(* Logix 5000 AddOnInstructionDefinition export IOLService; software revision 19.01 *)

TYPE IOLRequest :
STRUCT
   Enable_Multiple_Nodes : BOOL; {access None}   // Set to 1 to enable multiple nodes
   ApplicationPath : STRING; {access None}   // Set Path for following IOL Instructions
   Read : BOOL; {access None}   // For internal use to integrate IOLRead and IOWrite with IOLService
   Write : BOOL; {access None}   // For internal use to integrate IOLRead and IOWrite with IOLService
   Reset : BOOL; {access None}   // For internal use to integrate IOLRead and IOWrite with IOLService
   Done : BOOL; {access None}   // For internal use to integrate IOLRead and IOWrite with IOLService
   Error : BOOL; {access None}   // For internal use to integrate IOLRead and IOWrite with IOLService
   Slot : INT; {access None}   // For internal use to integrate IOLRead and IOWrite with IOLService
   Port : INT; {access None}   // For internal use to integrate IOLRead and IOWrite with IOLService
   Index : INT; {access None}   // For internal use to integrate IOLRead and IOWrite with IOLService
   SubIndex : INT; {access None}   // For internal use to integrate IOLRead and IOWrite with IOLService
   Length : INT; {access None}   // For internal use to integrate IOLRead and IOWrite with IOLService
   Handle : INT; {access None}   // For internal use to integrate IOLRead and IOWrite with IOLService
   Status : INT; {access None}   // For internal use to integrate IOLRead and IOWrite with IOLService
   NextHandle : INT; {access None}   // For internal use to integrate IOLRead and IOWrite with IOLService
   ReceiveData : SINT[145]; {access None}   // For internal use to integrate IOLRead and IOWrite with IOLService
   SendData : SINT[145]; {access None}   // For internal use to integrate IOLRead and IOWrite with IOLService
   WriteData : DINT; {access None}   // For internal use to integrate IOLRead and IOWrite with IOLService
   ActivePath : STRING; {access None}   // For internal use to integrate IOLRead and IOWrite with IOLService
END_STRUCT
END_TYPE

ADD_ON_INSTRUCTION IOLService   (* revision 1.2, ExecutePrescan *)
// Revision note:
// V1_0 Initial Release
// V1_1 Added error checking for IOLWrite operations
// V1_2 Added multiple EIP node support
// Help:
// IOL_Service - used with Turck BL20, BL67, BLC and TBEN IOLink masters to process requests from IOL_ReadString, IOL_WriteString, IOL_ReadData and IOL_WriteData AOI's.
// Status	Description
// 0	Operation completed successfully
// 	Status = 100 - 102, Ethernet IP MSG instruction errors - check communication parameters
// 100	IOL_SendMSG completed with error, check communication parameters
// 101	IOL_RecevieMSG completed with error, check communication parameters
// 110	IOL_Service Retry Limit exceeded
// 111	Slot specified not an IOLink master
// 	Status = 1000 to 1255, no response from device, connection error
// 1016	Device not connected or Port not configured as IOLink port
// 	Status = 2000 to 2255,  device response indicates error
// 2000	Device error, no details
// 2017	Device error, Index not available
// 2018	Device error, Subindex not available
// 2032	Device error, Service temporarily not available
// 2033	Device error, Service temporarily not available - local control
// 2034	Device error, Service temporarily not available - device control
// 2035	Device error, Index not writeable
// 2048	Device error, Parameter value out of range
// 2049	Device error, Parameter value above limit
// 2050	Device error, Parameter value below limit
// 2051	Device error, Parameter value length overrun (check IOLWrite precision/string length)
// 2052	Device error, Parameter value length underrun (check IOLWrite precision/string length)
// 2053	Device error, Function not available
// 2054	Device error, Function temporarily not available
// 2064	Device error, Parameter set invalid
// 2065	Device error, Inconsistent parameter set
// 2130	Device error, Application not ready
// 	Status = 3000 to 3255,   device response indicates vendor specific error
// 3000	Vendor specific error, no details
// 3001	Vendor specific error, vendor specific error number
// 3255	Vendor specific error, vendor specific error number
// 	Status = 7000 to 7255,  IOL-M Error Codes
// 7000	Unexpected write request instead of read request
// 7001	Decode error
// 7002	Port occupied by another task
// 	Status = 8000 to 8255,  IOL-M Error Codes
// 8000	Timeout when IOL-Ds or IOL-M ports are busy
// 8001	IOL Index out of range
// 8002	Port address greater than maximum
// 8003	Port function not supported
VAR_IN_OUT
   IOLData : IOLRequest; {required}
   IOL_SendMSG : MESSAGE; {required}
   IOL_ReceiveMSG : MESSAGE; {required}
END_VAR
VAR
   IOLS1 : BOOL;
   IOLS2 : BOOL;
   IOLS3 : BOOL;
   IOLS4 : BOOL;
   IOLS5 : BOOL;
   IOLS6 : BOOL;
   IOLS7 : BOOL;
   IOLReadActive : BOOL;
   IOLWriteActive : BOOL;
   Retry : BOOL;
   RetryCount : DINT;
   IOL_SendMSG_Request : BOOL; {access None}
   IOL_ReceiveMSG_Request : BOOL; {access None}
   IOLS4_Bad : BOOL; {access None}
   IOL_S2_0_Count : DINT; {access None}
   IOL_S6_0_Count : DINT; {access None}
   Busy_Retry : BOOL; {access None}
   IOL_S2_0_Total : DINT; {access None}
   IOL_S3_Retry : DINT; {access None}
   IOL_S1_Count : DINT; {access None}
   IOL_S2_Count : DINT; {access None}
   IOL_S3_Count : DINT; {access None}
   IOL_S5_Count : DINT; {access None}
   IOL_S6_Count : DINT; {access None}
   ER1 : BOOL; {access None}
   ER2 : BOOL; {access None}
   IOL_S6_NotBusy_Count : DINT; {access None}
   RetryTotal : DINT; {access None}
   IOL_S4_Bad_Count : DINT; {access None}
   IOL_S2_Error_Count : DINT; {access None}
   IOL_Done_Count : DINT; {access None}
   IOL_Error_Count : DINT; {access None}
   IOLReset_ONS : BOOL; {access None}
   ABS_RD_11 : INT; {access None}
   ABS_RD_12 : INT; {access None}
   ABS_RD_13 : INT; {access None}
   IOL_SendMSG_DN : BOOL; {access None}
   IOL_ReceiveMSG_DN : BOOL; {access None}
   IOLS2A : BOOL; {access None}
   Generate_Status : BOOL; {access None}
   IOLS5A : BOOL; {access None}
   Busy_Response : BOOL; {access None}
   Done_Response : BOOL; {access None}
   IOL_S6_Done_Count : DINT; {access None}
   Wait : BOOL; {access None}
   IOL_S6_Busy_Count : DINT; {access None}
END_VAR

ROUTINE Logic   (* ladder *)
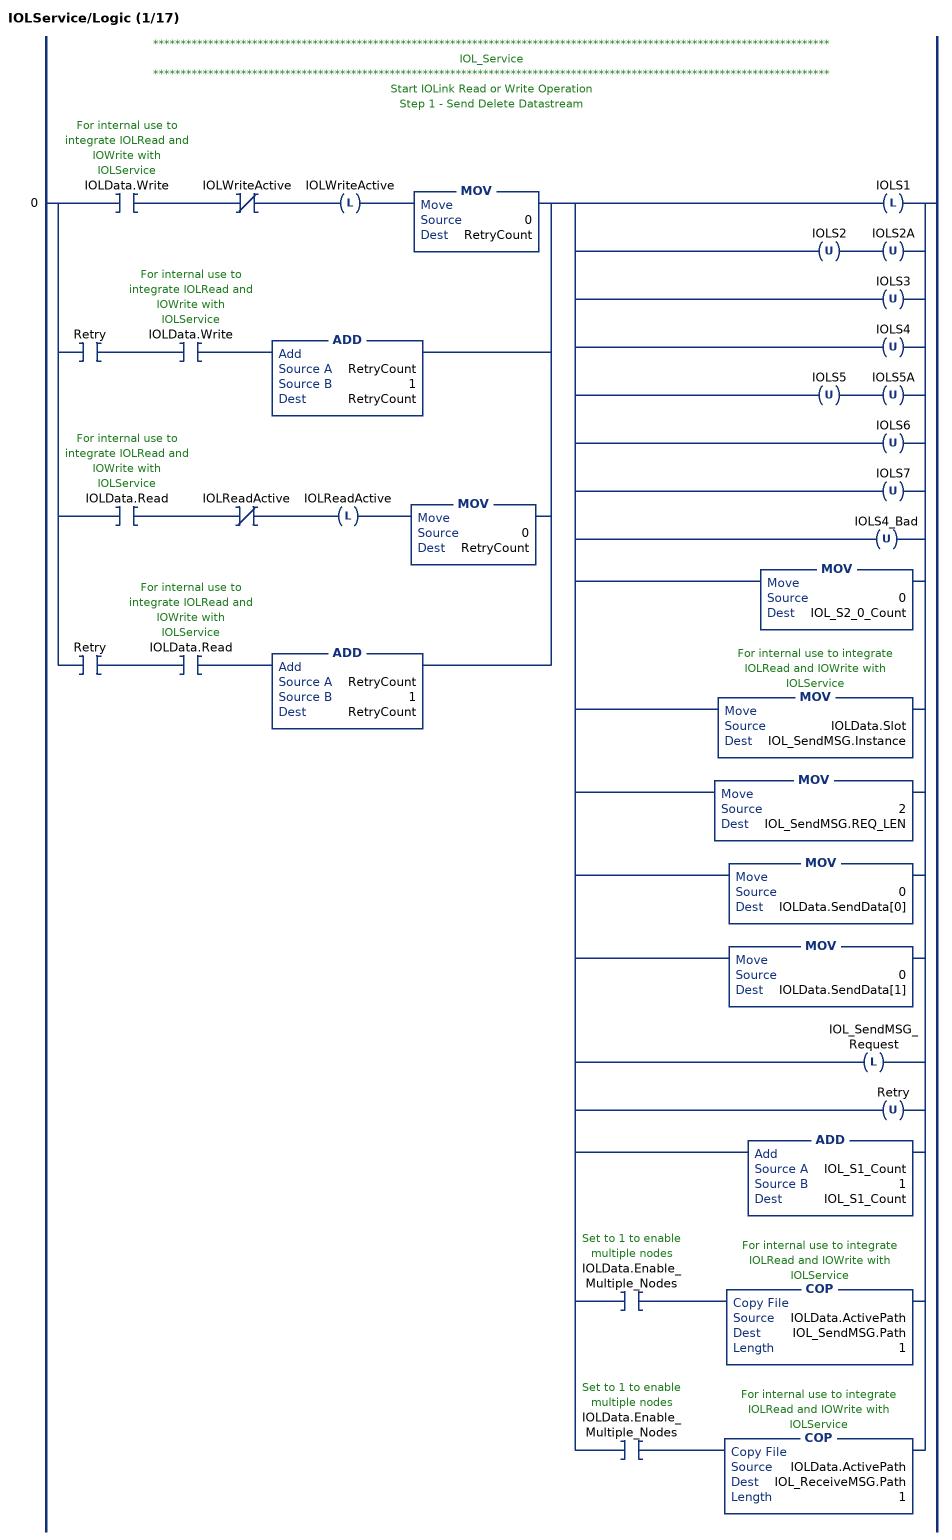
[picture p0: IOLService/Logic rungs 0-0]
   // ***************************************************************************************************************************
   // IOL_Service
   // ***************************************************************************************************************************
   // Start IOLink Read or Write Operation
   // Step 1 - Send Delete Datastream
   0: [XIC(IOLData.Write) XIO(IOLWriteActive) OTL(IOLWriteActive) MOV(0,RetryCount) ,XIC(Retry) XIC(IOLData.Write) ADD(RetryCount,1,RetryCount) ,XIC(IOLData.Read) XIO(IOLReadActive) OTL(IOLReadActive) MOV(0,RetryCount) ,XIC(Retry) XIC(IOLData.Read) ADD(RetryCount,1,RetryCount) ][OTL(IOLS1) ,OTU(IOLS2) OTU(IOLS2A) ,OTU(IOLS3) ,OTU(IOLS4) ,OTU(IOLS5) OTU(IOLS5A) ,OTU(IOLS6) ,OTU(IOLS7) ,OTU(IOLS4_Bad) ,MOV(0,IOL_S2_0_Count) ,MOV(IOLData.Slot,IOL_SendMSG.Instance) ,MOV(2,IOL_SendMSG.REQ_LEN) ,MOV(0,IOLData.SendData[0]) ,MOV(0,IOLData.SendData[1]) ,OTL(IOL_SendMSG_Request) ,OTU(Retry) ,ADD(IOL_S1_Count,1,IOL_S1_Count) ,XIC(IOLData.Enable_Multiple_Nodes) COP(IOLData.ActivePath,IOL_SendMSG.Path,1) ,XIC(IOLData.Enable_Multiple_Nodes) COP(IOLData.ActivePath,IOL_ReceiveMSG.Path,1) ];
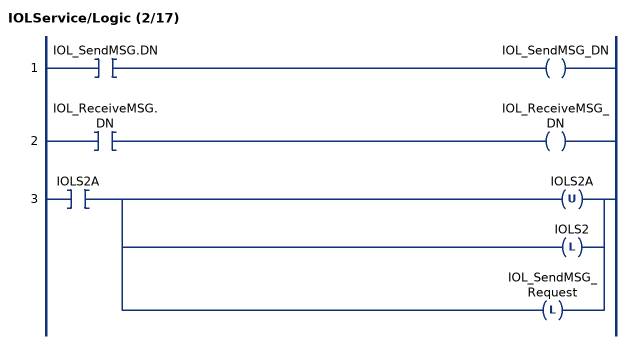
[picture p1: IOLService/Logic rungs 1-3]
   1: XIC(IOL_SendMSG.DN)OTE(IOL_SendMSG_DN);
   2: XIC(IOL_ReceiveMSG.DN)OTE(IOL_ReceiveMSG_DN);
   3: XIC(IOLS2A)[OTU(IOLS2A) ,OTL(IOLS2) ,OTL(IOL_SendMSG_Request) ];
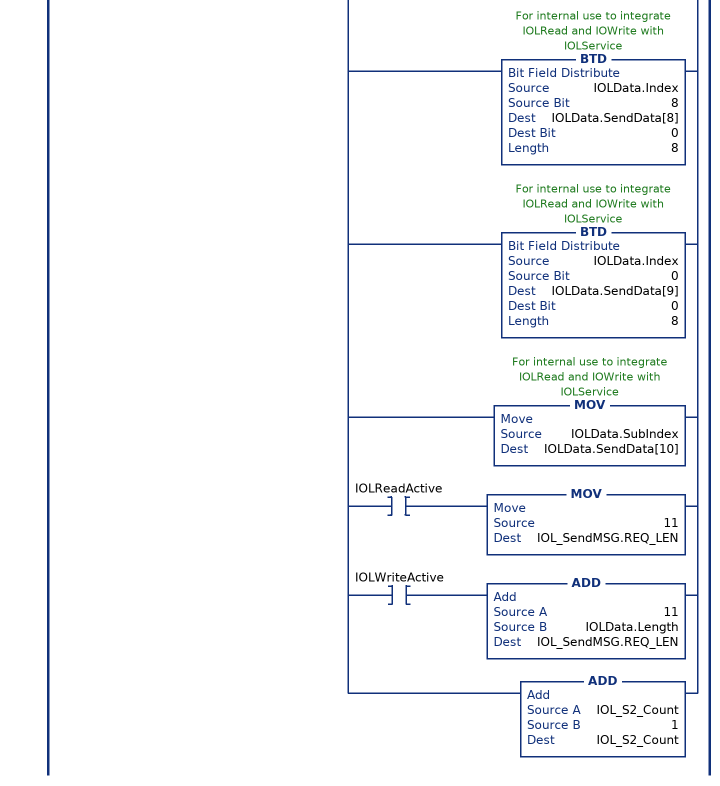
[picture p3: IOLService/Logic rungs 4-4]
   // Step 1 - After Delete Stream sent then Send IOLink Read or Write Request
   4: XIC(IOLS1)XIC(IOL_SendMSG_DN)XIO(IOL_SendMSG_Request)[OTU(IOLS1) ,OTL(IOLS2A) ,MOV(IOLData.Slot,IOL_SendMSG.Instance) ,MOV(0,IOLData.SendData[0]) ,MOV(16#fe,IOLData.SendData[1]) ,MOV(16#11,IOLData.SendData[2]) ,MOV(16#08,IOLData.SendData[3]) ,MOV(IOLData.Port,IOLData.SendData[4]) ,MOV(16#fe,IOLData.SendData[5]) ,MOV(16#4a,IOLData.SendData[6]) ,XIC(IOLReadActive) MOV(16#03,IOLData.SendData[7]) ,XIC(IOLWriteActive) MOV(16#02,IOLData.SendData[7]) ,BTD(IOLData.Index,8,IOLData.SendData[8],0,8) ,BTD(IOLData.Index,0,IOLData.SendData[9],0,8) ,MOV(IOLData.SubIndex,IOLData.SendData[10]) ,XIC(IOLReadActive) MOV(11,IOL_SendMSG.REQ_LEN) ,XIC(IOLWriteActive) ADD(11,IOLData.Length,IOL_SendMSG.REQ_LEN) ,ADD(IOL_S2_Count,1,IOL_S2_Count) ];
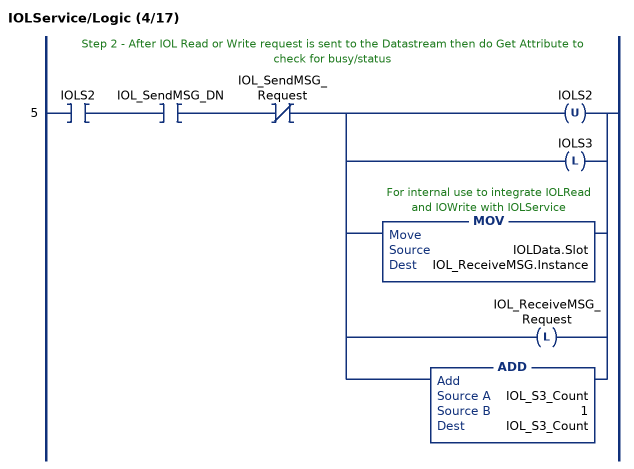
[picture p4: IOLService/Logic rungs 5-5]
   // Step 2 - After IOL Read or Write request is sent to the Datastream then do Get Attribute to check for busy/status
   5: XIC(IOLS2)XIC(IOL_SendMSG_DN)XIO(IOL_SendMSG_Request)[OTU(IOLS2) ,OTL(IOLS3) ,MOV(IOLData.Slot,IOL_ReceiveMSG.Instance) ,OTL(IOL_ReceiveMSG_Request) ,ADD(IOL_S3_Count,1,IOL_S3_Count) ];
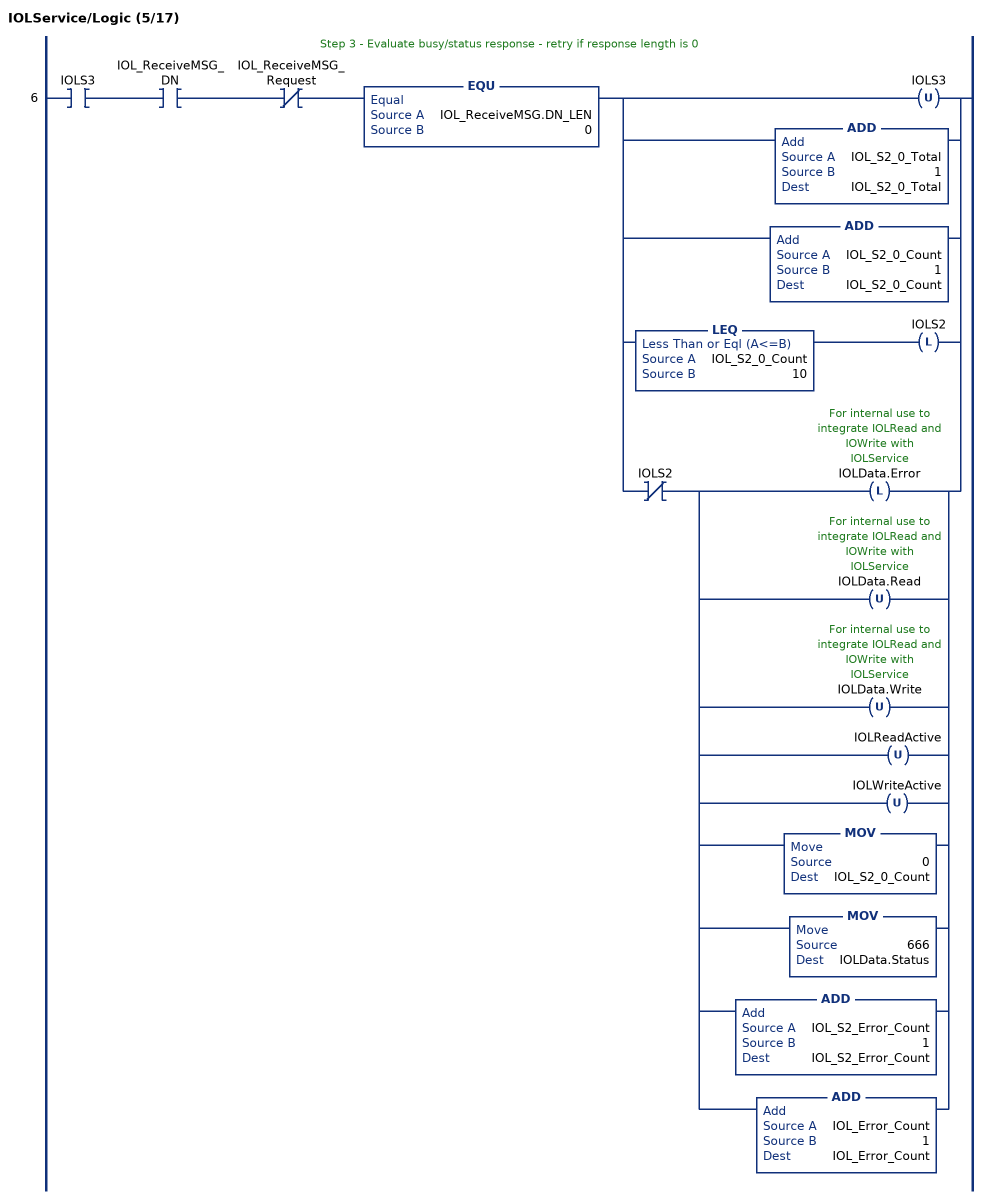
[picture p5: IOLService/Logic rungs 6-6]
   // Step 3 - Evaluate busy/status response - retry if response length is 0
   6: XIC(IOLS3)XIC(IOL_ReceiveMSG_DN)XIO(IOL_ReceiveMSG_Request)EQU(IOL_ReceiveMSG.DN_LEN,0)[OTU(IOLS3) ,ADD(IOL_S2_0_Total,1,IOL_S2_0_Total) ,ADD(IOL_S2_0_Count,1,IOL_S2_0_Count) ,LEQ(IOL_S2_0_Count,10) OTL(IOLS2) ,XIO(IOLS2) [OTL(IOLData.Error) ,OTU(IOLData.Read) ,OTU(IOLData.Write) ,OTU(IOLReadActive) ,OTU(IOLWriteActive) ,MOV(0,IOL_S2_0_Count) ,MOV(666,IOLData.Status) ,ADD(IOL_S2_Error_Count,1,IOL_S2_Error_Count) ,ADD(IOL_Error_Count,1,IOL_Error_Count) ] ];
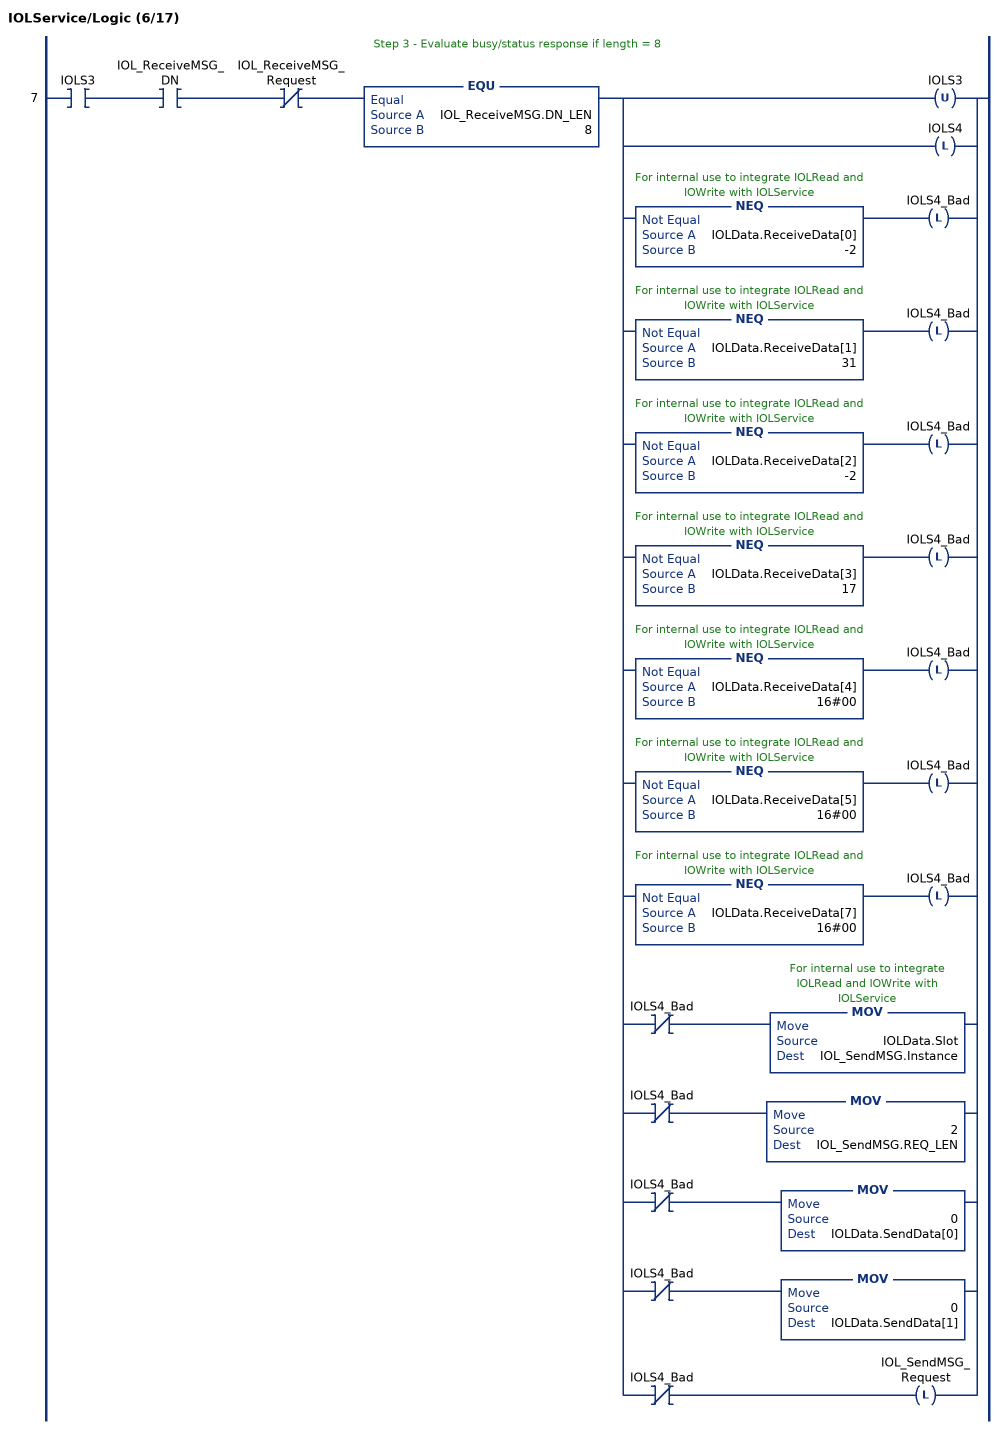
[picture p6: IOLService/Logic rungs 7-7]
   // Step 3 - Evaluate busy/status response if length = 8
   7: XIC(IOLS3)XIC(IOL_ReceiveMSG_DN)XIO(IOL_ReceiveMSG_Request)EQU(IOL_ReceiveMSG.DN_LEN,8)[OTU(IOLS3) ,OTL(IOLS4) ,NEQ(IOLData.ReceiveData[0],-2) OTL(IOLS4_Bad) ,NEQ(IOLData.ReceiveData[1],31) OTL(IOLS4_Bad) ,NEQ(IOLData.ReceiveData[2],-2) OTL(IOLS4_Bad) ,NEQ(IOLData.ReceiveData[3],17) OTL(IOLS4_Bad) ,NEQ(IOLData.ReceiveData[4],16#00) OTL(IOLS4_Bad) ,NEQ(IOLData.ReceiveData[5],16#00) OTL(IOLS4_Bad) ,NEQ(IOLData.ReceiveData[7],16#00) OTL(IOLS4_Bad) ,XIO(IOLS4_Bad) MOV(IOLData.Slot,IOL_SendMSG.Instance) ,XIO(IOLS4_Bad) MOV(2,IOL_SendMSG.REQ_LEN) ,XIO(IOLS4_Bad) MOV(0,IOLData.SendData[0]) ,XIO(IOLS4_Bad) MOV(0,IOLData.SendData[1]) ,XIO(IOLS4_Bad) OTL(IOL_SendMSG_Request) ];
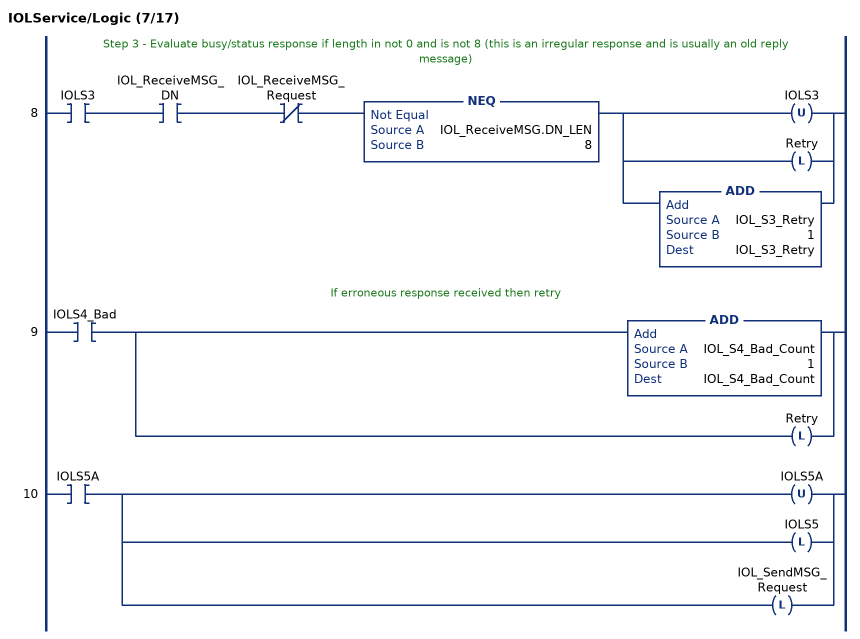
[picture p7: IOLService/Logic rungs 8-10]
   // Step 3 - Evaluate busy/status response if length in not 0 and is not 8 (this is an irregular response and is usually an old reply message)
   8: XIC(IOLS3)XIC(IOL_ReceiveMSG_DN)XIO(IOL_ReceiveMSG_Request)NEQ(IOL_ReceiveMSG.DN_LEN,8)[OTU(IOLS3) ,OTL(Retry) ,ADD(IOL_S3_Retry,1,IOL_S3_Retry) ];
   // If erroneous response received then retry
   9: XIC(IOLS4_Bad)[ADD(IOL_S4_Bad_Count,1,IOL_S4_Bad_Count) ,OTL(Retry) ];
   10: XIC(IOLS5A)[OTU(IOLS5A) ,OTL(IOLS5) ,OTL(IOL_SendMSG_Request) ];
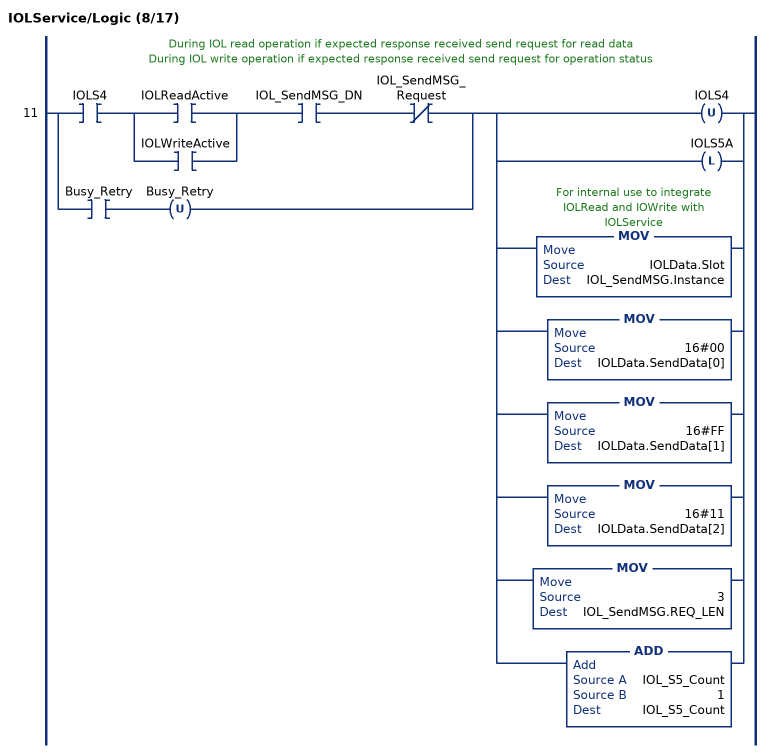
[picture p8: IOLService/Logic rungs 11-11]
   // During IOL read operation if expected response received send request for read data
   // During IOL write operation if expected response received send request for operation status
   11: [XIC(IOLS4) [XIC(IOLReadActive) ,XIC(IOLWriteActive) ] XIC(IOL_SendMSG_DN) XIO(IOL_SendMSG_Request) ,XIC(Busy_Retry) OTU(Busy_Retry) ][OTU(IOLS4) ,OTL(IOLS5A) ,MOV(IOLData.Slot,IOL_SendMSG.Instance) ,MOV(16#00,IOLData.SendData[0]) ,MOV(16#FF,IOLData.SendData[1]) ,MOV(16#11,IOLData.SendData[2]) ,MOV(3,IOL_SendMSG.REQ_LEN) ,ADD(IOL_S5_Count,1,IOL_S5_Count) ];
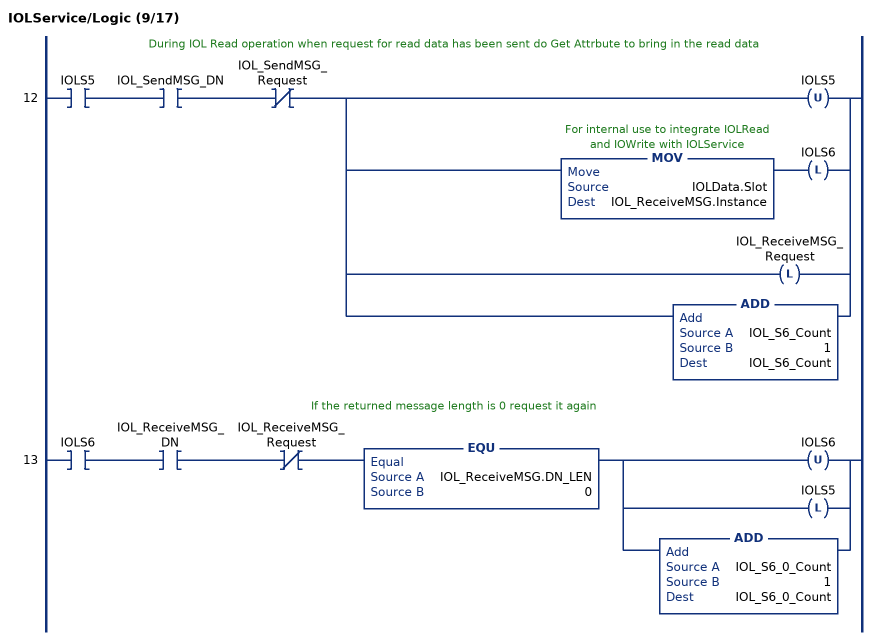
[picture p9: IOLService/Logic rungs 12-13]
   // During IOL Read operation when request for read data has been sent do Get Attrbute to bring in the read data
   12: XIC(IOLS5)XIC(IOL_SendMSG_DN)XIO(IOL_SendMSG_Request)[OTU(IOLS5) ,MOV(IOLData.Slot,IOL_ReceiveMSG.Instance) OTL(IOLS6) ,OTL(IOL_ReceiveMSG_Request) ,ADD(IOL_S6_Count,1,IOL_S6_Count) ];
   // If the returned message length is 0 request it again
   13: XIC(IOLS6)XIC(IOL_ReceiveMSG_DN)XIO(IOL_ReceiveMSG_Request)EQU(IOL_ReceiveMSG.DN_LEN,0)[OTU(IOLS6) ,OTL(IOLS5) ,ADD(IOL_S6_0_Count,1,IOL_S6_0_Count) ];
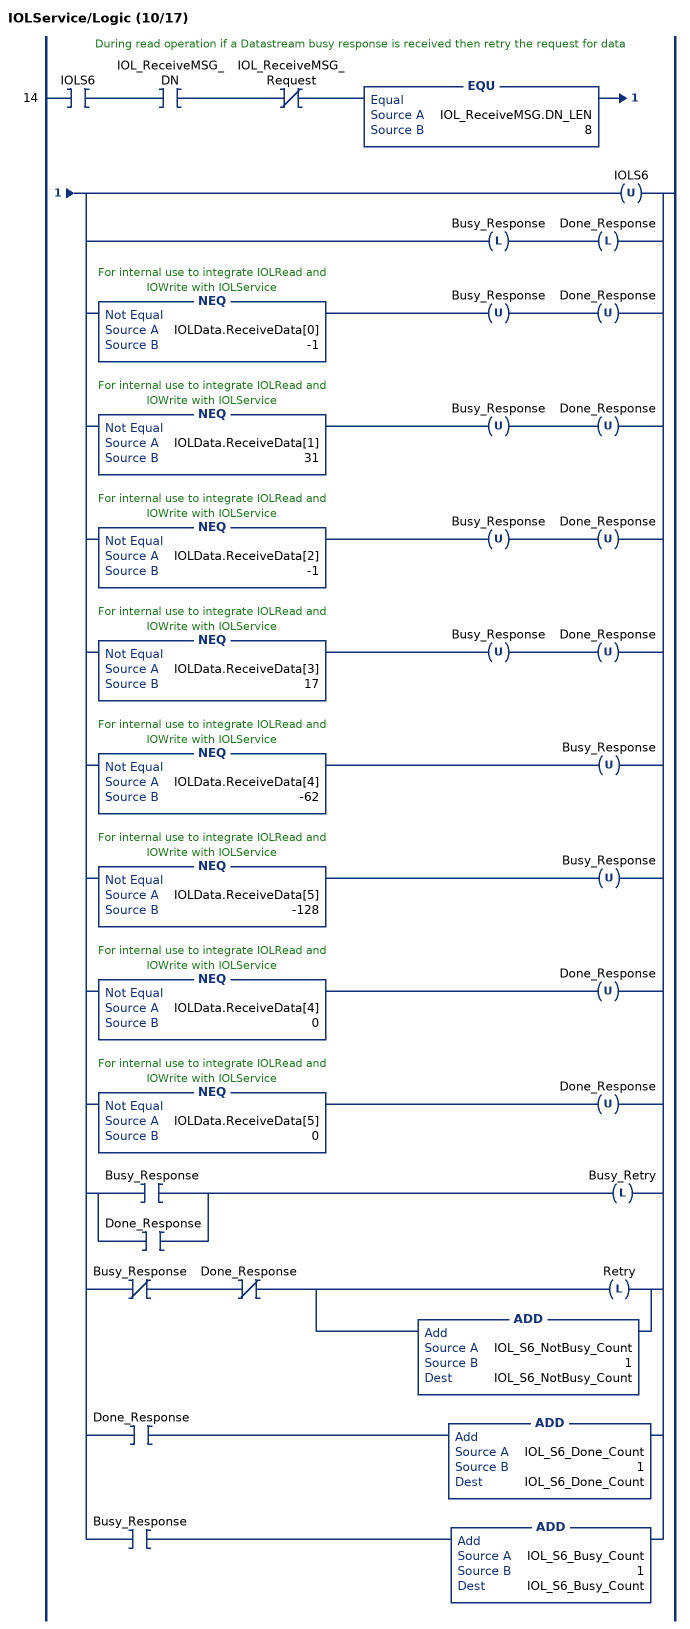
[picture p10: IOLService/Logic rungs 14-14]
   // During read operation if a Datastream busy response is received then retry the request for data
   14: XIC(IOLS6)XIC(IOL_ReceiveMSG_DN)XIO(IOL_ReceiveMSG_Request)EQU(IOL_ReceiveMSG.DN_LEN,8)[OTU(IOLS6) ,OTL(Busy_Response) OTL(Done_Response) ,NEQ(IOLData.ReceiveData[0],-1) OTU(Busy_Response) OTU(Done_Response) ,NEQ(IOLData.ReceiveData[1],31) OTU(Busy_Response) OTU(Done_Response) ,NEQ(IOLData.ReceiveData[2],-1) OTU(Busy_Response) OTU(Done_Response) ,NEQ(IOLData.ReceiveData[3],17) OTU(Busy_Response) OTU(Done_Response) ,NEQ(IOLData.ReceiveData[4],-62) OTU(Busy_Response) ,NEQ(IOLData.ReceiveData[5],-128) OTU(Busy_Response) ,NEQ(IOLData.ReceiveData[4],0) OTU(Done_Response) ,NEQ(IOLData.ReceiveData[5],0) OTU(Done_Response) ,[XIC(Busy_Response) ,XIC(Done_Response) ] OTL(Busy_Retry) ,XIO(Busy_Response) XIO(Done_Response) [OTL(Retry) ,ADD(IOL_S6_NotBusy_Count,1,IOL_S6_NotBusy_Count) ] ,XIC(Done_Response) ADD(IOL_S6_Done_Count,1,IOL_S6_Done_Count) ,XIC(Busy_Response) ADD(IOL_S6_Busy_Count,1,IOL_S6_Busy_Count) ];
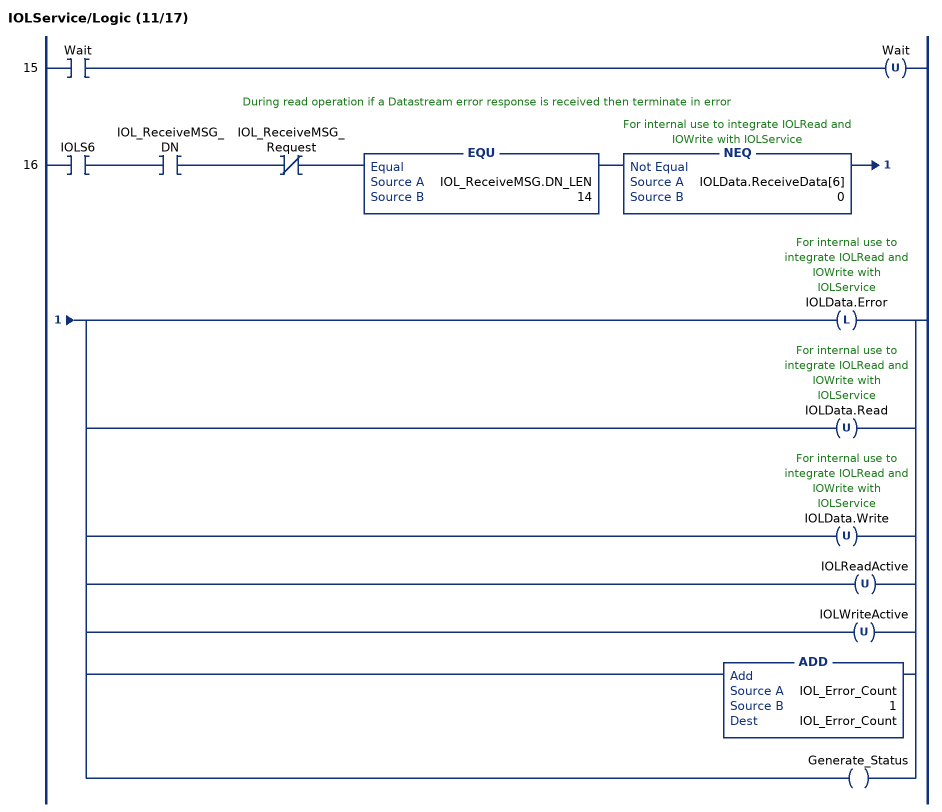
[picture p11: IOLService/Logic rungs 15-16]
   15: XIC(Wait)OTU(Wait);
   // During read operation if a Datastream error response is received then terminate in error
   16: XIC(IOLS6)XIC(IOL_ReceiveMSG_DN)XIO(IOL_ReceiveMSG_Request)EQU(IOL_ReceiveMSG.DN_LEN,14)NEQ(IOLData.ReceiveData[6],0)[OTL(IOLData.Error) ,OTU(IOLData.Read) ,OTU(IOLData.Write) ,OTU(IOLReadActive) ,OTU(IOLWriteActive) ,ADD(IOL_Error_Count,1,IOL_Error_Count) ,OTE(Generate_Status) ];
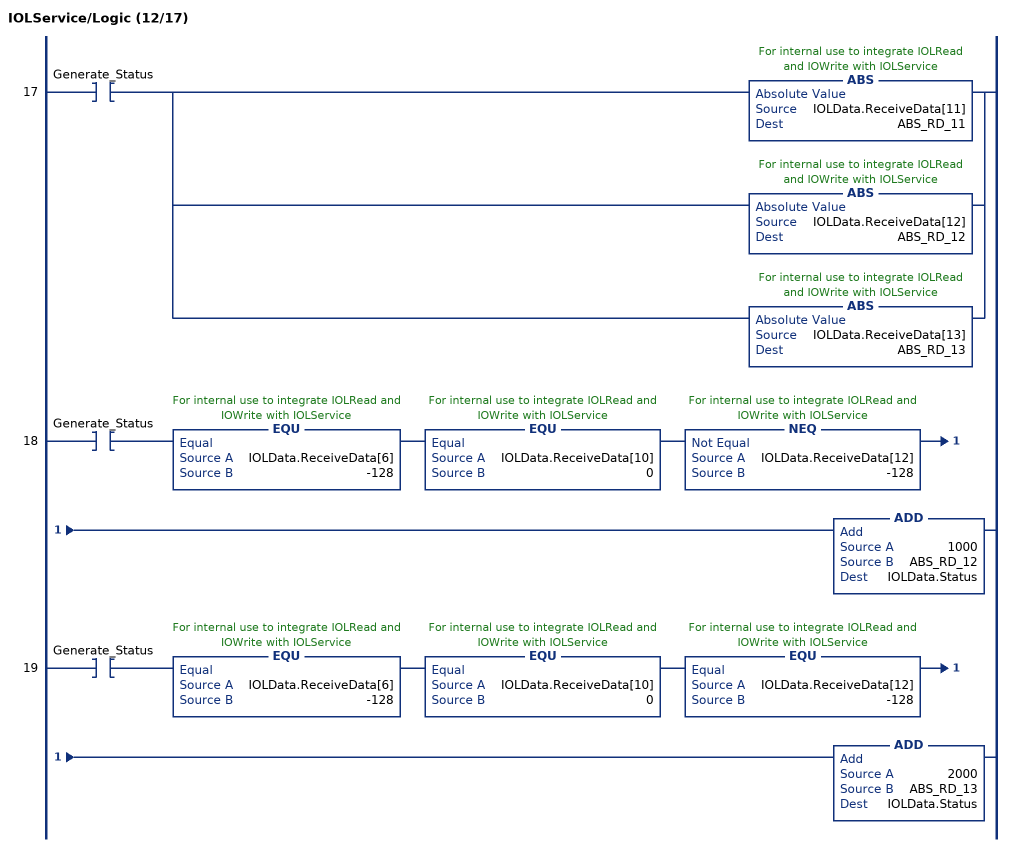
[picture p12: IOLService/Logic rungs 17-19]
   17: XIC(Generate_Status)[ABS(IOLData.ReceiveData[11],ABS_RD_11) ,ABS(IOLData.ReceiveData[12],ABS_RD_12) ,ABS(IOLData.ReceiveData[13],ABS_RD_13) ];
   18: XIC(Generate_Status)EQU(IOLData.ReceiveData[6],-128)EQU(IOLData.ReceiveData[10],0)NEQ(IOLData.ReceiveData[12],-128)ADD(1000,ABS_RD_12,IOLData.Status);
   19: XIC(Generate_Status)EQU(IOLData.ReceiveData[6],-128)EQU(IOLData.ReceiveData[10],0)EQU(IOLData.ReceiveData[12],-128)ADD(2000,ABS_RD_13,IOLData.Status);
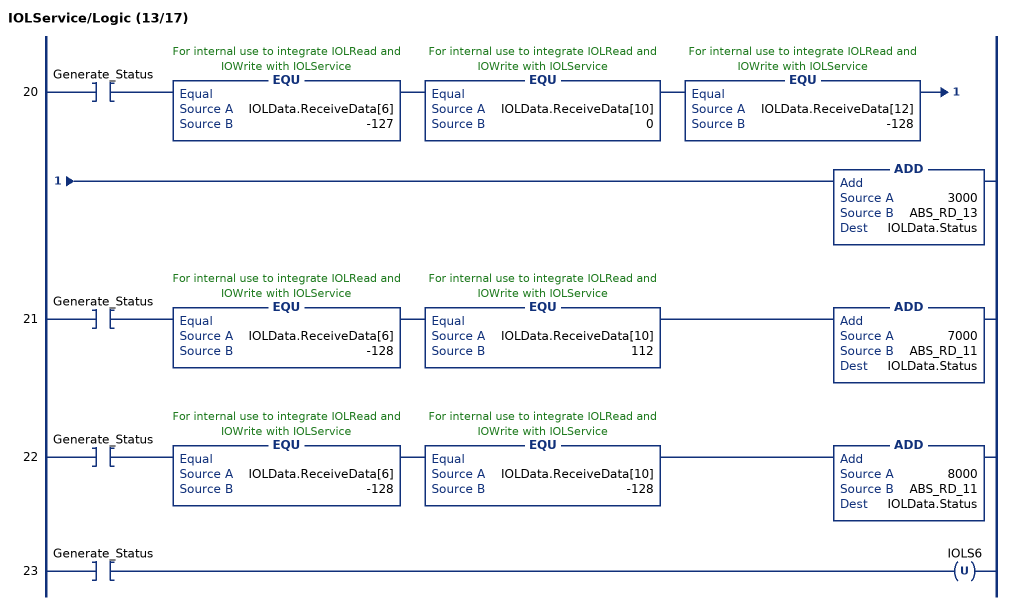
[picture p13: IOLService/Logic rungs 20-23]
   20: XIC(Generate_Status)EQU(IOLData.ReceiveData[6],-127)EQU(IOLData.ReceiveData[10],0)EQU(IOLData.ReceiveData[12],-128)ADD(3000,ABS_RD_13,IOLData.Status);
   21: XIC(Generate_Status)EQU(IOLData.ReceiveData[6],-128)EQU(IOLData.ReceiveData[10],112)ADD(7000,ABS_RD_11,IOLData.Status);
   22: XIC(Generate_Status)EQU(IOLData.ReceiveData[6],-128)EQU(IOLData.ReceiveData[10],-128)ADD(8000,ABS_RD_11,IOLData.Status);
   23: XIC(Generate_Status)OTU(IOLS6);
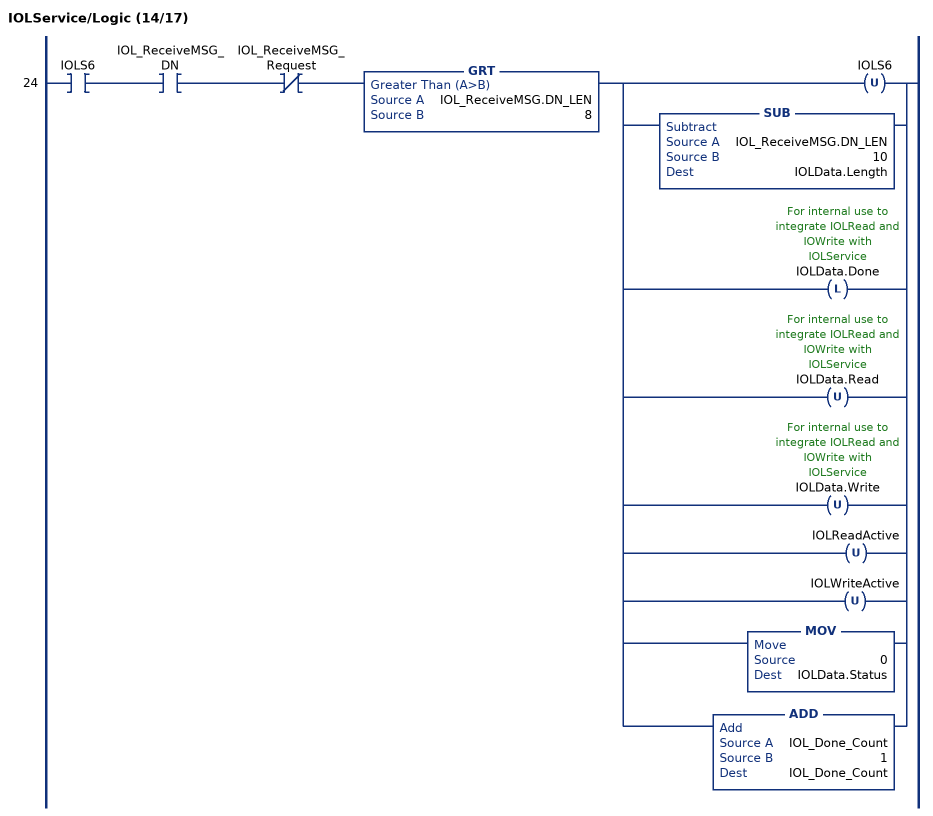
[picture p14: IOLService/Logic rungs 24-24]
   24: XIC(IOLS6)XIC(IOL_ReceiveMSG_DN)XIO(IOL_ReceiveMSG_Request)GRT(IOL_ReceiveMSG.DN_LEN,8)[OTU(IOLS6) ,SUB(IOL_ReceiveMSG.DN_LEN,10,IOLData.Length) ,OTL(IOLData.Done) ,OTU(IOLData.Read) ,OTU(IOLData.Write) ,OTU(IOLReadActive) ,OTU(IOLWriteActive) ,MOV(0,IOLData.Status) ,ADD(IOL_Done_Count,1,IOL_Done_Count) ];
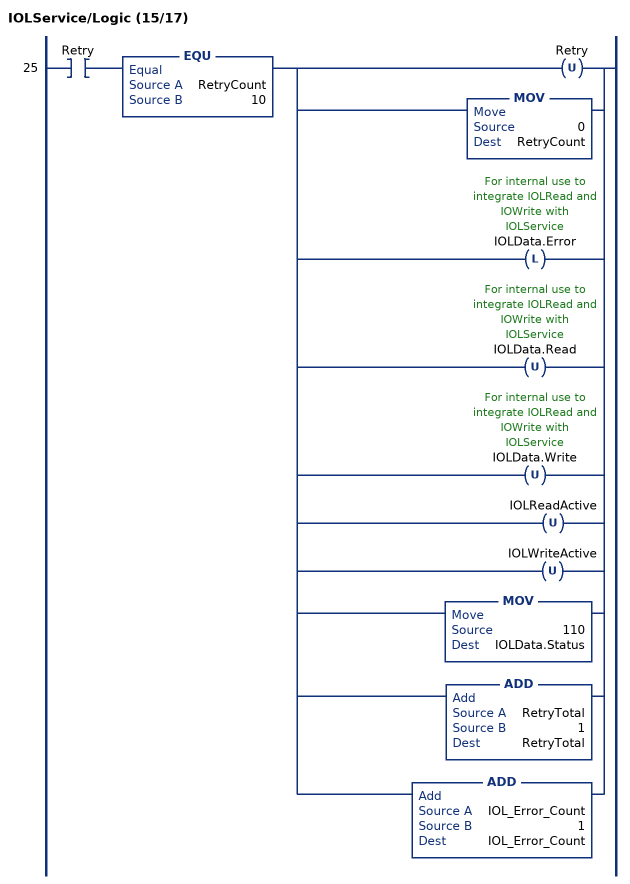
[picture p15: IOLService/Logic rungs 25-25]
   25: XIC(Retry)EQU(RetryCount,10)[OTU(Retry) ,MOV(0,RetryCount) ,OTL(IOLData.Error) ,OTU(IOLData.Read) ,OTU(IOLData.Write) ,OTU(IOLReadActive) ,OTU(IOLWriteActive) ,MOV(110,IOLData.Status) ,ADD(RetryTotal,1,RetryTotal) ,ADD(IOL_Error_Count,1,IOL_Error_Count) ];
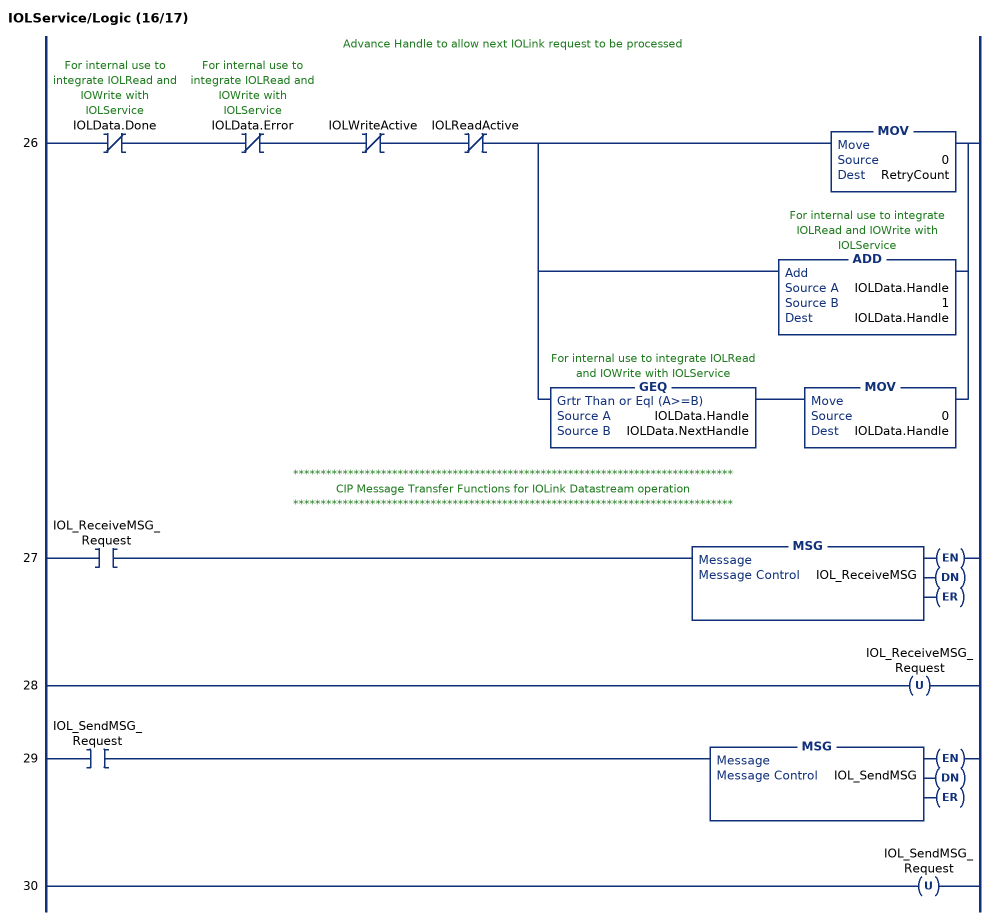
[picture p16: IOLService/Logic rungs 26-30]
   // Advance Handle to allow next IOLink request to be processed
   26: XIO(IOLData.Done)XIO(IOLData.Error)XIO(IOLWriteActive)XIO(IOLReadActive)[MOV(0,RetryCount) ,ADD(IOLData.Handle,1,IOLData.Handle) ,GEQ(IOLData.Handle,IOLData.NextHandle) MOV(0,IOLData.Handle) ];
   // ********************************************************************************
   // CIP Message Transfer Functions for IOLink Datastream operation
   // ********************************************************************************
   27: XIC(IOL_ReceiveMSG_Request)MSG(IOL_ReceiveMSG);
   28: OTU(IOL_ReceiveMSG_Request);
   29: XIC(IOL_SendMSG_Request)MSG(IOL_SendMSG);
   30: OTU(IOL_SendMSG_Request);
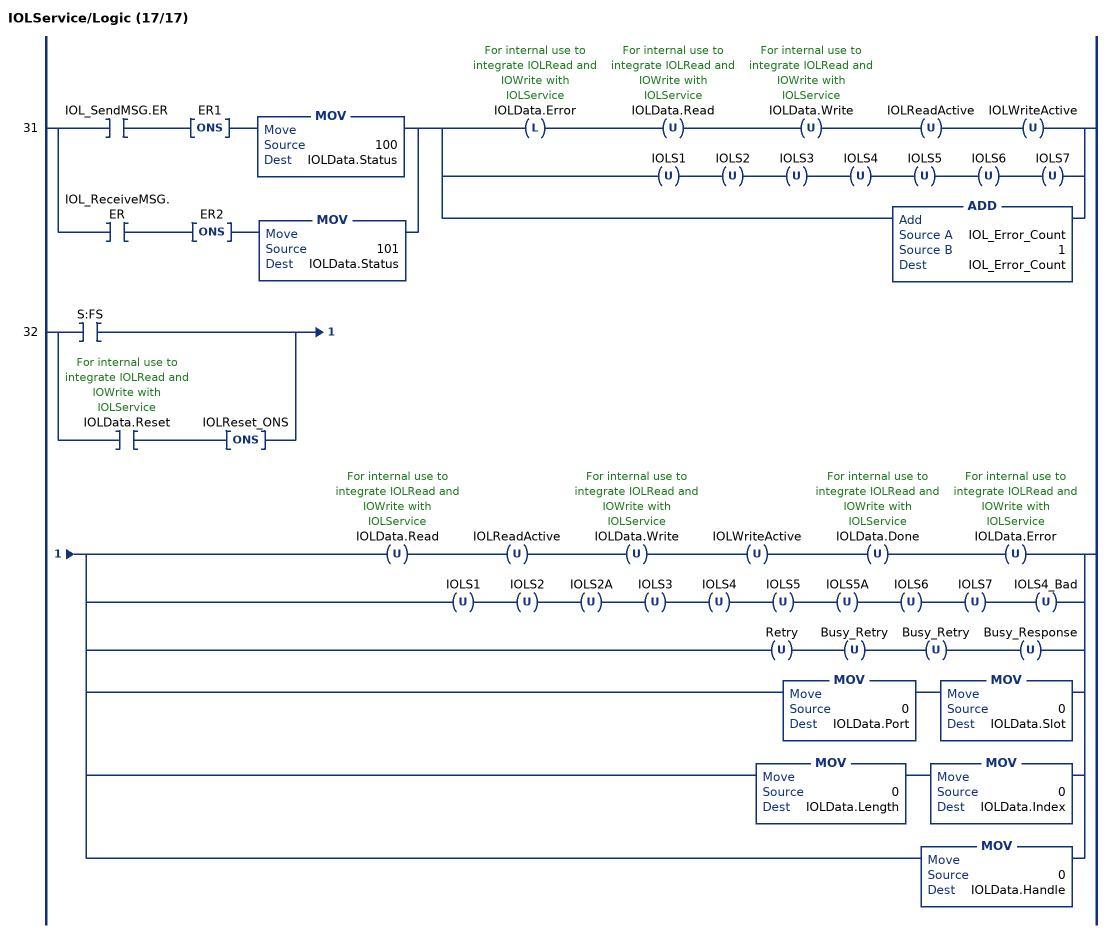
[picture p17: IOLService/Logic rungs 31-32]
   31: [XIC(IOL_SendMSG.ER) ONS(ER1) MOV(100,IOLData.Status) ,XIC(IOL_ReceiveMSG.ER) ONS(ER2) MOV(101,IOLData.Status) ][OTL(IOLData.Error) OTU(IOLData.Read) OTU(IOLData.Write) OTU(IOLReadActive) OTU(IOLWriteActive) ,OTU(IOLS1) OTU(IOLS2) OTU(IOLS3) OTU(IOLS4) OTU(IOLS5) OTU(IOLS6) OTU(IOLS7) ,ADD(IOL_Error_Count,1,IOL_Error_Count) ];
   32: [XIC(S:FS) ,XIC(IOLData.Reset) ONS(IOLReset_ONS) ][OTU(IOLData.Read) OTU(IOLReadActive) OTU(IOLData.Write) OTU(IOLWriteActive) OTU(IOLData.Done) OTU(IOLData.Error) ,OTU(IOLS1) OTU(IOLS2) OTU(IOLS2A) OTU(IOLS3) OTU(IOLS4) OTU(IOLS5) OTU(IOLS5A) OTU(IOLS6) OTU(IOLS7) OTU(IOLS4_Bad) ,OTU(Retry) OTU(Busy_Retry) OTU(Busy_Retry) OTU(Busy_Response) ,MOV(0,IOLData.Port) MOV(0,IOLData.Slot) ,MOV(0,IOLData.Length) MOV(0,IOLData.Index) ,MOV(0,IOLData.Handle) ];
END_ROUTINE

ROUTINE Prescan   (* ladder *)
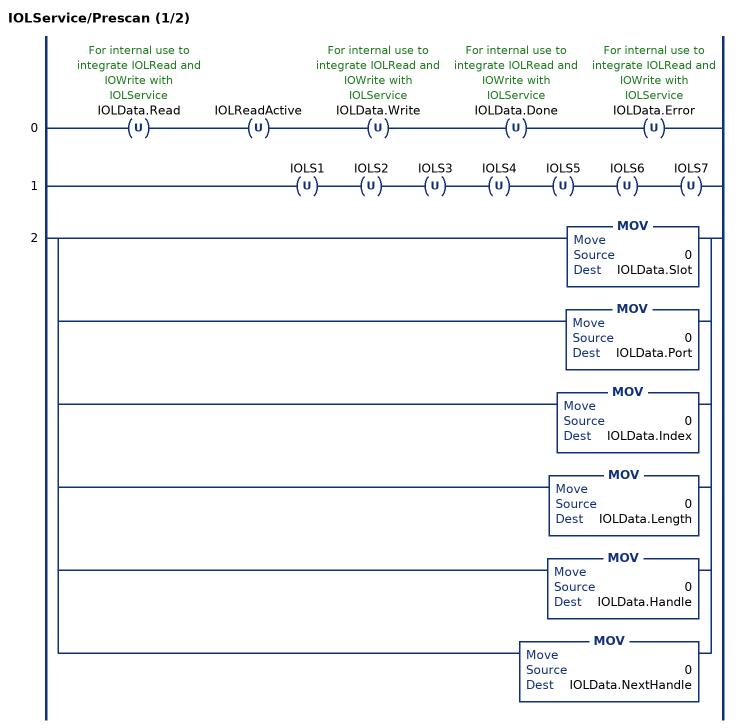
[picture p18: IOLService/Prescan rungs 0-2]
   0: OTU(IOLData.Read)OTU(IOLReadActive)OTU(IOLData.Write)OTU(IOLData.Done)OTU(IOLData.Error);
   1: OTU(IOLS1)OTU(IOLS2)OTU(IOLS3)OTU(IOLS4)OTU(IOLS5)OTU(IOLS6)OTU(IOLS7);
   2: [MOV(0,IOLData.Slot) ,MOV(0,IOLData.Port) ,MOV(0,IOLData.Index) ,MOV(0,IOLData.Length) ,MOV(0,IOLData.Handle) ,MOV(0,IOLData.NextHandle) ];
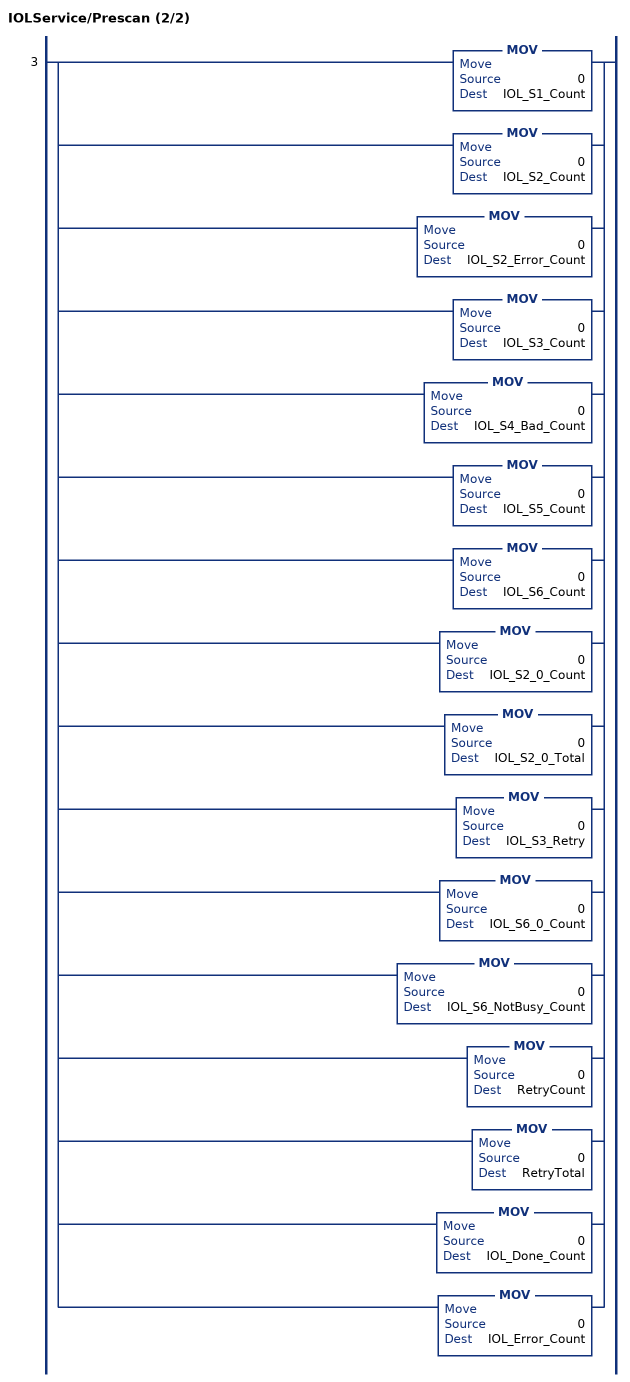
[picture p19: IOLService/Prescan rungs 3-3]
   3: [MOV(0,IOL_S1_Count) ,MOV(0,IOL_S2_Count) ,MOV(0,IOL_S2_Error_Count) ,MOV(0,IOL_S3_Count) ,MOV(0,IOL_S4_Bad_Count) ,MOV(0,IOL_S5_Count) ,MOV(0,IOL_S6_Count) ,MOV(0,IOL_S2_0_Count) ,MOV(0,IOL_S2_0_Total) ,MOV(0,IOL_S3_Retry) ,MOV(0,IOL_S6_0_Count) ,MOV(0,IOL_S6_NotBusy_Count) ,MOV(0,RetryCount) ,MOV(0,RetryTotal) ,MOV(0,IOL_Done_Count) ,MOV(0,IOL_Error_Count) ];
END_ROUTINE
END_ADD_ON_INSTRUCTION
